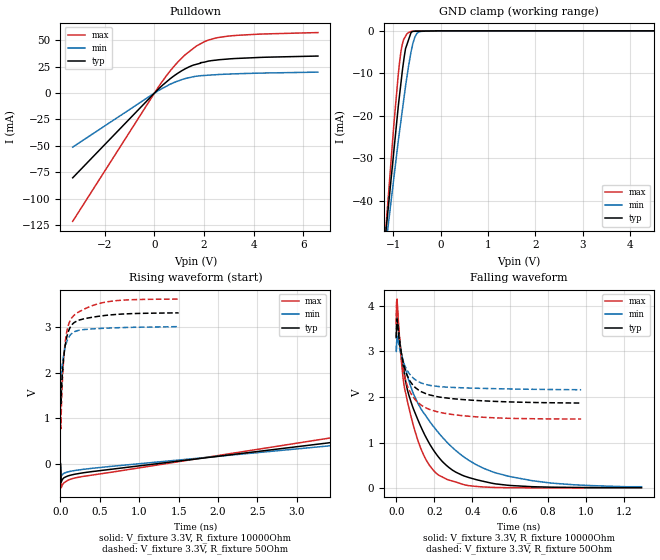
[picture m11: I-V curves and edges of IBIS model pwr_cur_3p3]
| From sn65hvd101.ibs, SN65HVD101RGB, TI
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|   pwr_cur_3p3 Model
[Model]   pwr_cur_3p3
Model_type   Open_drain
Polarity   Inverting
Vmeas = 1.65
Vref = 3.3
Cref = 2pF
Rref = 10000
|   typ   min   max
|   (nom PVT)   (fast PVT)   (slow PVT)
C_comp   1.553e-12   1.546e-12   1.553e-12
| Where nom  PVT is Nominal Process, 3.3V, 45C
|   Fast PVT is Strong Process,  3.6V, -20C
|   Slow PVT is Weak Process,   3V, 125C
[Voltage Range]   3.3   3   3.6
|Junction Temperature
[Temperature Range]   45   125   -20
[Pullup Reference]   3.3   3   3.6
[Pulldown Reference]   0   0   0
[Power Clamp Reference]   3.3   3   3.6
[GND Clamp Reference]   0   0   0
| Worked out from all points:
|   slope of the pulldown table from 0 to 0.495 V, typ, clamps not added: 45.8 ohm
|   GND clamp passes 1 mA (typ) near -0.65 V on its own axis
|   falling waveform, V_fixture 3.3V, R_fixture 10000Ohm: 20-80 % time 187ps typ, 314ps min, 120ps max; typ from 3.3 V to 0.014 V
|   rising waveform, V_fixture 3.3V, R_fixture 10000Ohm: 20-80 % time 28.2ns typ, 29.6ns min, 27.8ns max; typ from 0.014 V to 3.3 V
|   falling waveform, V_fixture 3.3V, R_fixture 50Ohm: 20-80 % time 92.4ps typ, 89.5ps min, 82.8ps max; typ from 3.3 V to 1.87 V
|   rising waveform, V_fixture 3.3V, R_fixture 50Ohm: 20-80 % time 101ps typ, 95.9ps min, 111ps max; typ from 1.86 V to 3.3 V
[Pulldown]
|   Voltage   I(typ)   I(min)   I(max)
-3.3V     -80.33mA   -51.22mA   -121.6mA
262.8mV   6.047mA    3.708mA    9.302mA
630mV     13.49mA    8.343mA    20.88mA
939.6mV   18.77mA    11.33mA    29.32mA
1.246V    23.05mA    13.79mA    36.43mA
1.688V    27.25mA    15.99mA    44.49mA
2.167V    30.27mA    16.94mA    50.15mA
2.473V    31.22mA    17.42mA    52.18mA
2.934V    32.22mA    17.97mA    53.87mA
4.162V    33.7mA     18.86mA    55.8mA
6.6V      35.11mA    19.86mA    57.36mA
[GND Clamp]
|   Voltage   I(typ)   I(min)   I(max)
-3.3V     -292.9mA   -257.4mA   -347.1mA
-1.214V   -53.31mA   -55.35mA   -54.63mA
-1.141V   -45.07mA   -48.52mA   -43.52mA
-993.6mV  -28.44mA   -34.75mA   -22.25mA
-867.6mV  -14.72mA   -23.27mA   -7.035mA
-817.2mV  -9.853mA   -19.05mA   -3.337mA
-745.8mV  -4.213mA   -13.06mA   -1.283mA
-630mV    -446.2uA   -5.018mA   -162.9uA
-549mV    -112.4uA   -1.492mA   -56.18uA
-507mV    -103.8uA   -630.6uA   -35.01uA
-285mV    -58.03uA   -2.197uA   -419.7nA
6.6V      0A         0A         0A
[POWER Clamp]
|   Voltage   I(typ)   I(min)   I(max)
-3.3V     0A         0A         0A
0V        0A         0A         0A
6.6V      0A         0A         0A
[Ramp]
R_load = 10000
|   typ   min   max
dV/dt_r   1.97006/2.8121e-08   1.78619/2.94368e-08   2.15236/2.76877e-08
dV/dt_f   1.97172/1.87485e-10   1.78688/3.17585e-10   2.15417/1.19543e-10
[Falling Waveform]
V_fixture = 3.3V
V_fixture_min = 3V
V_fixture_max = 3.6V
R_fixture = 10000Ohm
|   Time   V(typ)   V(min)   V(max)
0s        3.3V       3V         3.6V
2ps       3.614V     3.193V     4.09V
4ps       3.73V      3.311V     4.145V
36ps      2.689V     2.803V     2.413V
90ps      1.745V     2.076V     1.376V
150ps     1.17V      1.621V     679mV
218ps     708.7mV    1.24V      304.9mV
346ps     289.3mV    717.7mV    93.24mV
526ps     95.39mV    336mV      17.81mV
1.292ns   14.44mV    34.47mV    9.712mV
[Rising Waveform]
V_fixture = 3.3V
V_fixture_min = 3V
V_fixture_max = 3.6V
R_fixture = 10000Ohm
|   Time   V(typ)   V(min)   V(max)
0s        13.57mV    19.48mV    9.726mV
10ps      -388.3mV   -261.3mV   -512.2mV
90ps      -255.7mV   -165.7mV   -350.7mV
280ps     -186.2mV   -110.5mV   -264.6mV
4.59ns    680.7mV    575.1mV    813.6mV
16.14ns   1.806V     1.58V      2.017V
26.36ns   2.398V     2.123V     2.653V
38.79ns   2.815V     2.517V     3.094V
71.15ns   3.204V     2.899V     3.502V
132.5ns   3.3V       3V         3.6V
[Falling Waveform]
V_fixture = 3.3V
V_fixture_min = 3V
V_fixture_max = 3.6V
R_fixture = 50Ohm
|   Time   V(typ)   V(min)   V(max)
0s        3.3V       3V         3.6V
2ps       3.606V     3.189V     4.077V
4ps       3.703V     3.295V     4.104V
14ps      3.324V     3.134V     3.423V
24ps      3.022V     2.946V     2.963V
54ps      2.508V     2.61V      2.298V
90ps      2.249V     2.413V     1.997V
144ps     2.095V     2.291V     1.788V
394ps     1.932V     2.196V     1.574V
974ps     1.868V     2.159V     1.517V
[Rising Waveform]
V_fixture = 3.3V
V_fixture_min = 3V
V_fixture_max = 3.6V
R_fixture = 50Ohm
|   Time   V(typ)   V(min)   V(max)
0s        1.861V     2.15V      1.516V
2ps       1.495V     1.974V     1.001V
4ps       1.322V     1.868V     771.7mV
16ps      1.72V      2.036V     1.442V
28ps      2.055V     2.233V     1.922V
60ps      2.586V     2.553V     2.653V
104ps     2.911V     2.764V     3.053V
178ps     3.094V     2.891V     3.257V
614ps     3.253V     2.97V      3.547V
1.5ns     3.3V       3V         3.6V
